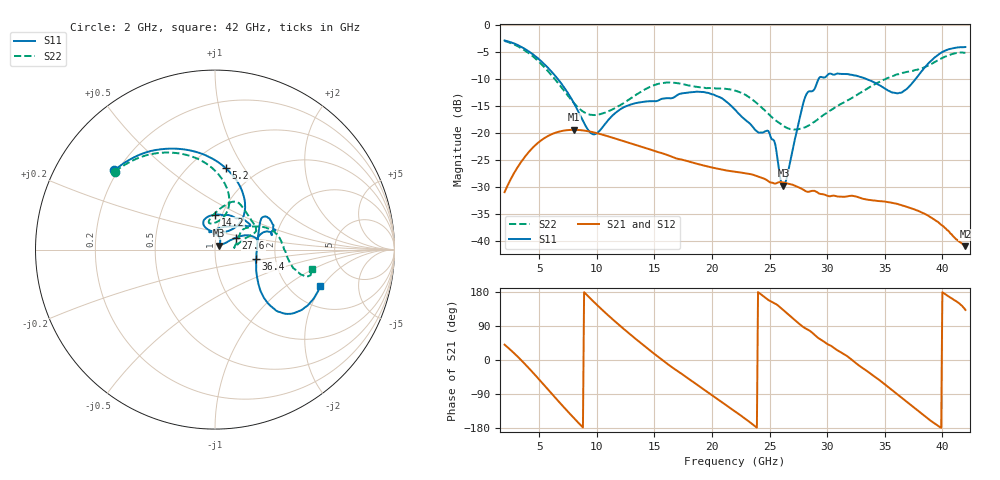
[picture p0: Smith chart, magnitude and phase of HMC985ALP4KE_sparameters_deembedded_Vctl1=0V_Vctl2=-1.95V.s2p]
!s2p File: Measurements: S11, S21, S12, S22
# GHz S dB R 50.0
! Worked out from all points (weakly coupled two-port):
!   401 points, 2 GHz to 42 GHz, reference 50 ohm
!   highest |S21| = -19.41 dB at 8 GHz (marker M1); lowest = -40.9 dB at 42 GHz (marker M2)
!   lowest |S11| = -29.7 dB at 26.2 GHz (marker M3), VSWR 1.07, Z = 52.3 + j2.38 ohm
!   |S11| at or under -10 dB: 6.604 GHz to 29.27 GHz (22.66 GHz wide, 126 % of centre); 33.36 GHz to 37.7 GHz (4.331 GHz wide, 12.2 % of centre)
!   |S22| runs from -19.4 to -3.0 dB; largest |S21 - S12| = 0.00022
!   S11 on the Smith chart (normalised r, x): 2 GHz: 0.19, +0.34; 5.2 GHz: 0.73, +0.83; 14.2 GHz: 0.93, +0.38; 27.6 GHz: 1.25, +0.17; 36.4 GHz: 1.58, -0.18; 42 GHz: 2.90, -1.91
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2  -2.93 141.8  -30.91 40.4  -30.91 40.4  -3.02 142.1
3.6  -4.30 112.6  -24.85 -5.4  -24.85 -5.4  -4.57 114.0
5.2  -6.81 82.3  -21.31 -58.3  -21.32 -58.3  -7.32 88.7
8  -14.43 47.0  -19.41 -152.7  -19.42 -152.8  -14.43 74.9
8.7  -17.34 52.2  -19.50 -174.9  -19.50 -174.9  -15.89 82.8
9.9  -20.18 90.0  -19.97 148.8  -19.97 148.8  -16.67 98.4
12.1  -15.56 113.0  -21.35 88.2  -21.35 88.2  -14.79 96.5
14.2  -14.21 89.7  -22.74 35.4  -22.75 35.4  -11.93 77.4
15.4  -13.94 73.1  -23.58 7.0  -23.58 7.0  -10.91 69.5
19.3  -12.46 34.4  -26.01 -77.7  -26.01 -77.7  -11.64 40.6
22  -15.69 52.3  -27.14 -135.3  -27.15 -135.3  -12.18 23.6
25  -20.08 98.4  -29.06 156.6  -29.06 156.6  -16.69 16.5
26.2  -29.72 44.0  -29.14 131.1  -29.14 131.1  -18.70 8.6
27.6  -17.41 29.6  -30.09 94.8  -30.09 94.8  -19.24 7.0
28.1  -13.33 20.9  -30.69 83.6  -30.68 83.5  -18.94 10.2
28.7  -12.29 12.9  -30.67 72.2  -30.68 72.2  -18.21 15.7
31  -9.06 23.3  -31.73 23.8  -31.74 23.7  -14.88 35.0
33.3  -9.94 34.2  -32.22 -25.9  -32.23 -25.8  -12.07 30.9
35.4  -12.27 12.2  -32.79 -73.5  -32.80 -73.6  -9.75 20.4
36.4  -12.58 -13.0  -33.27 -97.9  -33.29 -98.0  -8.98 14.0
39.5  -5.81 -43.4  -36.26 -171.1  -36.28 -171.4  -6.72 -14.0
42  -4.14 -19.0  -40.88 132.1  -40.89 132.3  -5.19 -11.4
